[IBIS Ver]  4.0
[File Name]lpc3131_0_3v_tfbga180.ibs
[File Rev]  1.0
[Date]  2010 Jan 25 (Mon) 11:58:19
[Source]  Package model from Ansoft Q3D Extractor 7.1.1
[Notes]   IO models Rev 0.20 IBIS Model Design Automation Generation
[Copyright]  NXP Semiconductors. All rights reserved.
|   LPC3131/LPC3130_TFBGA180 (180 TFBGA package) IBIS Model
[Disclaimer]
| NXP Semiconductors warrants and represents that the IBIS models
| identified herein are owned by NXP Semiconductors (NXP).  The
| models provided are not warranted as fully representing all of the
| operating characteristics and specifications of the semiconductor
| products to which the models relate.  Moreover, unless there is a
| signed, written agreement to the contrary, these models are furnished
| on an "as is" basis without support or warranty of any kind, either
| expressed or implied, regarding the use thereof, and NXP
| specifically disclaims all implied warranties of merchantability and
| fitness of the models for any purpose.
| NXP does not assume any liability arising out of the application
| or use of these IBIS models including infringement of patents and
| copyrights, nor does NXP convey any license under its patents and
| copyrights or the rights of others.
| NXP provides IBIS models as a service to our customers.  You and
| your company shall not distribute, convey, sell, or give these models
| to anyone else without receiving prior written permission from
| NXP.
[Component]   LPC3131_0_TFBGA180
[Manufacturer]  NXP
[Package]
|   typ   min   max
R_pkg   115.08m   5.63m   297.68m
L_pkg   2.91nH   0.70nH   5.41nH
C_pkg   1.35pF   0.51pF   2.38pF
| IMPORTANT NOTES:
| This model is valid for the following part types:
| LPC3131
| LPC3130
| Pins follow the groupings in the data sheet
| Pad name definitions
| APIO - Analog pad input output
[Pin]   signal_name   model_name   | comments
|   CLOCK GENERATION SIGNALS
A10   FFAST_IN   NC   | APIO pads not modeled
B10   FFAST_OUT   NC   | APIO pads not modeled
D11   VDDA12   POWER   | PLL_OSC supply
E10   VDDA12   POWER   | PLL_OSC supply
E9   VSSA12   gnd   | PLL_OSC gnd
H14   RSTIN_N   NC   | Hard wired to be in only
H12   CLK_256FS_O   bspts3chp
J4   CLOCK_OUT   bspts3chp
G13   SYSCLK_O   bspts3chp
|   10-BIT ADC SIGNALS
A13   ADC10B_VDDA33   POWER   |10-bit ADC Analog Supply
A12   ADC10B_GNDA   POWER   |10-bit ADC Analog gnd
B14   ADC10B_GPA0   NC   |apio3v3 10-bit ADC Analog Input
A14   ADC10B_GPA1   NC   |apio3v3 10-bit ADC Analog Input
B13   ADC10B_GPA2   NC   |apio3v3 10-bit ADC Analog Input
C14   ADC10B_GPA3   NC   |apio3v3 10-bit ADC Analog Input
|   USB HS 2.0 OTG
L2   USB_VBUS   NC   |apiot5v USB supply detection line
M1   USB_ID   NC   |apio3v3
J5   USB_RREF   NC   |apio3v3
P2   USB_DP   NC   |apio3v3 USB D+
N2   USB_DM   NC   |apio3v3 USB D-
L1   USB_VDDA12_PLL   POWER   |USB PLL supply
M2   USB_VDDA33_DRV   POWER   |USB Analog supply for driver
P1   USB_VDDA33   POWER   |USB Analog supply for PHY
L3   USB_VSSA_TERM   gnd   |
N1   USB_GNDA   gnd   |CG1 USB Analog gnd
K4   USB_VSSA_REF   gnd   |CG1 USB Analog gnd
|   JTAG
N11   JTAGSEL   bspts3chp   |JTAG selection.
K9   TDI   bspts3chp   |JTAG Data Input
P13   TRST_N   bspts3chp   |JTAG Reset Input
M14   TCK   bspts3chp   |JTAG Clock Input
P10   TMS   bspts3chp   |JTAG Mode Select Input
F10   SCAN_TDO   bspts3chp   |JTAG TDO
E11   ARM_TDO   bspts3chp   |JTAG TDO
F11   BUF_TRST_N   bspts3chp   |Buffered TRST_N out signal
D13   BUF_TCK   bspts3chp   |Buffered TCK out signal.
D14   BUF_TMS   bspts3chp   |Buffered TMS out signal.
|   UART
N13   mUART_CTS_NA   bspts3chp   |UART Clear To Send
P14   mUART_RTS_N   bspts3chp   |UART Ready To Send
P12   UART_RXD   bspts3chp   |UART Serial Input
N12   UART_TXD   bspts3chp   |UART Serial Output
|   I2C
C10   I2C_SDA0   iic3m4sdat5v_400k   |I2C Data Line
D10   I2C_SCL0   iic3m4sclt5v_400k   |I2C Clock line
E12   I2C_SDA1   bspts3chp   |I2C Data Line
E13   I2C_SCL1   bspts3chp   |I2C Clock line
|   SPI
A7   SPI_CS_OUT0   mem1bsptz40pch   |SPI Chip Select
A8   SPI_SCK   mem1bsptz40pch   |SPI Clock Input
C8   SPI_MISO   mem1bsptz40pch   |SPI Data Input
B7   SPI_MOSI   mem1bsptz40pch   |SPI Data Output
B8   SPI_CS_IN   mem1bsptz40pch   |SPI Chip Select Input
|VDDI
H3   VDDI   POWER
L7   VDDI   POWER
L12   VDDI   POWER
C12   VDDI   POWER
C6   VDDI   POWER
|VSSI
A11   VSSI   gnd
C7   VSSI   gnd
D12   VSSI   gnd
G4   VSSI   gnd
L6   VSSI   gnd
L11   VSSI   gnd
|VDDE_IOA
B2   VDDE_IOA   POWER
E5   VDDE_IOA   POWER
F5   VDDE_IOA   POWER
G5   VDDE_IOA   POWER
H5   VDDE_IOA   POWER
|VDDE_IOB
L4   VDDE_IOB   POWER
M5   VDDE_IOB   POWER
M7   VDDE_IOB   POWER
M9   VDDE_IOB   POWER
|VDDE_IOC
C13   VDDE_IOC   POWER
D5   VDDE_IOC   POWER
D7   VDDE_IOC   POWER
E8   VDDE_IOC   POWER
G12   VDDE_IOC   POWER
L10   VDDE_IOC   POWER
|VSSE_IOA
C3   VSSE_IOA   gnd
C4   VSSE_IOA   gnd
E4   VSSE_IOA   gnd
F4   VSSE_IOA   gnd
H4   VSSE_IOA   gnd
K3   VSSE_IOA   gnd
|VSSE_IOB
M3   VSSE_IOB   gnd
M4   VSSE_IOB   gnd
M6   VSSE_IOB   gnd
M8   VSSE_IOB   gnd
|   LCD INTERFACE
K8   mLCD_CSB   mem1bsptz40pch   |LCD Chip Select
L8   mLCD_E_RD   mem1bsptz40pch   |LCD 6800 En 8080 Rd En
P8   mLCD_RS   mem1bsptz40pch   |LCD Inst Register
N9   mLCD_RW_WR   mem1bsptz40pch   |LCD 6800 Rd/wr slct
N8   mLCD_DB_0   mem1bsptz40pch   |LCD Data 0
P9   mLCD_DB_1   mem1bsptz40pch   |LCD Data 1
N6   mLCD_DB_2   mem1bsptz40pch   |LCD Data 2
P6   mLCD_DB_3   mem1bsptz40pch   |LCD Data 3
N7   mLCD_DB_4   mem1bsptz40pch   |LCD Data 4
P7   mLCD_DB_5   mem1bsptz40pch   |LCD Data 5
K6   mLCD_DB_6   mem1bsptz40pch   |LCD Data 6
P5   mLCD_DB_7   mem1bsptz40pch   |LCD Data 7
N5   mLCD_DB_8   mem1bsptz40pch   |LCD Data 8
L5   mLCD_DB_9   mem1bsptz40pch   |LCD Data 9
K7   mLCD_DB_10   mem1bsptz40pch   |LCD Data 10
N4   mLCD_DB_11   mem1bsptz40pch   |LCD Data 11
K5   mLCD_DB_12   mem1bsptz40pch   |LCD Data 12
P4   mLCD_DB_13   mem1bsptz40pch   |LCD Data 13
P3   mLCD_DB_14   mem1bsptz40pch   |LCD Data 14
N3   mLCD_DB_15   mem1bsptz40pch   |LCD Data 15
|I2S/Digital Audio Input
M10   I2SRX_DATA0   bspts3chp   |I2S Serial Data Receive Inpt
G14   I2SRX_DATA1   bspts3chp   |I2S Serial Data Receive Inpt
N10   I2SRX_BCK0   bspts3chp   |I2S Bitclock
F14   I2SRX_BCK1   bspts3chp   |I2S Bitclock
P11   I2SRX_WS0   bspts3chp   |I2S Word select
F13   I2SRX_WS1   bspts3chp   |I2S Word select
|I2S/Digital Audio Output
M13   mI2STX_DATA0   bspts3chp   |I2S Serial Data Transmit Ou
M12   mI2STX_BCK0   bspts3chp   |I2S Bitclock
M11   mI2STX_WS0   bspts3chp   |I2S Word select
N14   mI2STX_CLK0   bspts3chp   |I2S Serial Clock
F12   I2STX_DATA1   bspts3chp   |I2S Serial Data Transmit Out
E14   I2STX_BCK1   bspts3chp   |I2S Bitclock
G10   I2STX_WS1   bspts3chp   |I2S Word select
|General Purpose IO
K10   GPIO0   bspts3chp   |General Purpose IO Pin 0
J10   GPIO1   bspts3chp   |General Purpose IO Pin 1
L14   GPIO2   bspts3chp   |General Purpose IO Pin 2
B11   GPIO3   bspts3chp   |General Purpose IO Pin 3
C11   GPIO4   bspts3chp   |General Purpose Input Pin 4
B6   mGPIO5   mem1bsptz40pch   |General Purpose IO Pin 5
A6   mGPIO6   mem1bsptz40pch   |General Purpose IO Pin 6
A5   mGPIO7   mem1bsptz40pch   |General Purpose IO Pin 7
B5   mGPIO8   mem1bsptz40pch   |General Purpose IO Pin 8
C5   mGPIO9   mem1bsptz40pch   |General Purpose IO Pin 9
A4   mGPIO10   mem1bsptz40pch   |General Purpose IO Pin 10
H13   GPIO11   bspts3chp   |General Purpose IO Pin 11
H10   GPIO12   bspts3chp   |General Purpose IO Pin 12
J12   GPIO13   bspts3chp   |General Purpose IO Pin 13
J14   GPIO14   bspts3chp   |General Purpose IO Pin 14
J13   GPIO15   bspts3chp   |General Purpose IO Pin 15
J11   GPIO16   bspts3chp   |General Purpose IO Pin 16
K12   GPIO17   bspts3chp   |General Purpose IO Pin 17
K14   GPIO18   bspts3chp   |General Purpose IO Pin 18
H11   GPIO19   bspts3chp   |General Purpose IO Pin 19
K13   GPIO20   bspts3chp   |General Purpose IO Pin 20
|External Bus Interface (NAND flash controller)
B3   EBI_A_0_ALE   mem1bsptz40pch   |EBI Address Latch Enable
A2   EBI_A_1_CLE   mem1bsptz40pch   |EBI Command Latch Enable
G2   EBI_D_0   mem1bsptz40pch   |EBI Data I/O 0
F2   EBI_D_1   mem1bsptz40pch   |EBI Data I/O 1
F1   EBI_D_2   mem1bsptz40pch   |EBI Data I/O 2
E1   EBI_D_3   mem1bsptz40pch   |EBI Data I/O 3
E2   EBI_D_4   mem1bsptz40pch   |EBI Data I/O 4
D1   EBI_D_5   mem1bsptz40pch   |EBI Data I/O 5
D2   EBI_D_6   mem1bsptz40pch   |EBI Data I/O 6
C1   EBI_D_7   mem1bsptz40pch   |EBI Data I/O 7
B1   EBI_D_8   mem1bsptz40pch   |EBI Data I/O 8
A3   EBI_D_9   mem1bsptz40pch   |EBI Data I/O 9
A1   EBI_D_10   mem1bsptz40pch   |EBI Data I/O 10
C2   EBI_D_11   mem1bsptz40pch   |EBI Data I/O 11
G3   EBI_D_12   mem1bsptz40pch   |EBI Data I/O 12
D3   EBI_D_13   mem1bsptz40pch   |EBI Data I/O 13
E3   EBI_D_14   mem1bsptz40pch   |EBI Data I/O 14
F3   EBI_D_15   mem1bsptz40pch   |EBI Data I/O 15
H1   EBI_DQM_0_NOE   mem1bsptz40pch   |NAND Rd En active low)
J2   EBI_NWE   mem1bsptz40pch   |NAND W En (active low)
J1   NAND_NCS_0   mem1bsptz40pch   |NAND Chip Enable 0
J3   NAND_NCS_1   mem1bsptz40pch   |NAND Chip Enable 1
K1   NAND_NCS_2   mem1bsptz40pch   |NAND Chip Enable 2
K2   NAND_NCS_3   mem1bsptz40pch   |NAND Chip Enable 3
E6   mNAND_RYBN0   mem1bsptz40pch   |NAND Ready/Busy 0
E7   mNAND_RYBN1   mem1bsptz40pch   |NAND Ready/Busy 1
B4   mNAND_RYBN2   mem1bsptz40pch   |NAND Ready/Busy 2
D4   mNAND_RYBN3   mem1bsptz40pch   |NAND Ready/Busy 3
G1   EBI_NCAS_BLOUT_0  mem1bsptz40pch   |EBI Lower lane byte select
H2   EBI_NRAS_BLOUT_1  mem1bsptz40pch   |EBI Upper lane byte select
|Pulse Width Modulation module
B9   PWM_DATA   bspts3chp   |PWM Output
[Model Selector] mem1bsptz40pch
m1bsptz40pchp_p_hs   Plain input Mode (esh=0 p1=0, p2=1)
m1bsptz40pchp_p_ls   Plain input Mode (esh=1 p1=0, p2=1)
m1bsptz40pchp_pd_hs   Pull Down Mode (esh=0 p1=1, p2=1)
m1bsptz40pchp_pd_ls   Pull Down Mode (esh=1 p1=1, p2=1)
m1bsptz40pchp_pu_hs   Pull Up Mode (esh=0 p1=0, p2=0)
m1bsptz40pchp_pu_ls   Pull Up Mode (esh=1 p1=0, p2=0)
m1bsptz40pchp_r_hs   Repeater Mode (esh=0 p1=1, p2=0)
m1bsptz40pchp_r_ls   Repeater Mode (esh=1 p1=1, p2=0)
[Model Selector] bspts3chp
bspts3chp_p   Plain input Mode (p1=0, p2=1)
bspts3chp_pd   Pull Down Mode (p1=1, p2=1)
bspts3chp_pu   Pull Up Mode (p1=0, p2=0)
bspts3chp_r   Repeater Mode (p1=1, p2=0)
| Models and submodels in the file (14): iic3m4sclt5v_400k (I/O_open_drain), iic3m4sdat5v_400k (I/O_open_drain), m1bsptz40pchp_pd_hs (I/O), m1bsptz40pchp_pd_ls (I/O), m1bsptz40pchp_p_hs (I/O), m1bsptz40pchp_p_ls (I/O), m1bsptz40pchp_pu_hs (I/O), m1bsptz40pchp_pu_ls (I/O), m1bsptz40pchp_r_hs (I/O), m1bsptz40pchp_r_ls (I/O), bspts3chp_p (I/O), bspts3chp_pd (I/O), bspts3chp_pu (I/O), bspts3chp_r (I/O)
